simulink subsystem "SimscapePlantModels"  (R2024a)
settings: Solver=VariableStepAuto  StartTime=0.0  StopTime=10.0  RelTol=1e-3
undefined symbols (not defined in the file or in its folder): PlntTrnsfrCaseAxlSpdLock, PlntTrnsfrCaseTrqSplitRatio
libraries: simulink x2, nesl_utility x2

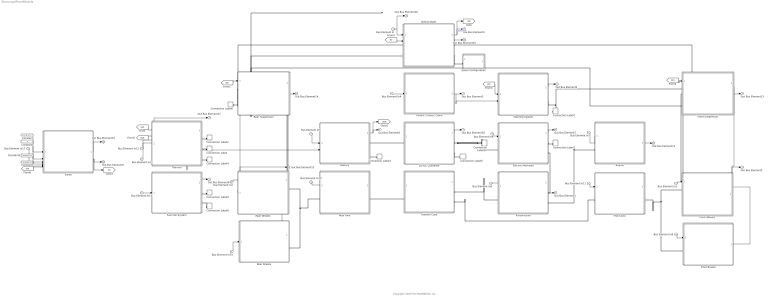
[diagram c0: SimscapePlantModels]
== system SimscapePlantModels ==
  note: Copyright 2023 The MathWorks, Inc.
  Bus Element In{,1..3} (4 alike) : Inport
  Bus Element In4 : Inport  Port=2
  Bus Element In{5..14,17} (11 alike) : Inport  Port=3
  Battery : Subsystem  Variant=on  VariantChoicesSpecifier={'BatteryMappedSSC', 'DetailedBatteryModel', 'NoBattery'}  VariantControlMode=label  VariantControl=Battery  LabelModeActiveChoice=NoBattery
  Connection Label : ConnectionLabel  Label=ThrmEM
  Connection Label1 : ConnectionLabel  Label=ThrmEM
  Connection Label10 : ConnectionLabel  Label=HVDC
  Connection Label2 : ConnectionLabel  Label=ThrmBatt
  Connection Label3 : ConnectionLabel  Label=ThrmBatt
  Connection Label4 : ConnectionLabel  Label=ThrmPwrE
  Connection Label5 : ConnectionLabel  Label=ThrmPwrE
  Connection Label6 : ConnectionLabel  Label=Steer
  Connection Label7 : ConnectionLabel  Label=Steer
  Connection Label8 : ConnectionLabel  Label=ThrmPwrE
  Connection Label9 : ConnectionLabel  Label=HVDC
  Constant : Constant  Value=[0 0 0 0 0 0]
  Constant1 : Constant  Value=0
  Constant3 : Constant  Value=zeros(2,1)
  Constant4 : Constant  Value=ones(2,1)
  DC-DC Converter : Subsystem  Variant=on  VariantChoicesSpecifier={'DCDCConverterSSC', 'HVDCPassThroughSSC', 'NoDCDCConverter'}  VariantControlMode=label  VariantControl=DC-DC Converter  LabelModeActiveChoice=NoDCDCConverter
  Electric Machines : Subsystem  Variant=on  VariantChoicesSpecifier={'s1EMSSC', 's2EMSSC', 's3EMSSC', 's4EMSSC', 'NoEM'}  VariantControlMode=label  VariantControl=Electric Machines  LabelModeActiveChoice=NoEM
  Engine : Subsystem  Variant=on  VariantChoicesSpecifier={'FMUEngineSSC', 'NoEngine', 'SimpleEngineSSC'}  VariantControlMode=label  VariantControl=Engine  LabelModeActiveChoice=SimpleEngineSSC
  Front Axle : Subsystem  Variant=on  VariantChoicesSpecifier={'DualEMDriveFrontSSC', 'LimitedSlipDifferentialSSC', 'NoDifferentialFrontSSC', 'OpenDifferentialSSC'}  VariantControlMode=label  VariantControl=Front Axle  LabelModeActiveChoice=OpenDifferentialSSC
  Front Brakes : Subsystem  Variant=on  VariantControlMode=label  LabelModeActiveChoice=BrakingHydraulicsDiscBrakesFrontSSC
  Front Suspension : Subsystem  Variant=on  VariantChoicesSpecifier={'NoSuspensionFrontSSC', 'MultibodySuspensionFrontSSC'}  VariantControlMode=label  VariantControl=Front Suspension  LabelModeActiveChoice=NoSuspensionFrontSSC
  Front Wheels : Subsystem  Variant=on  VariantChoicesSpecifier={'MFTiresLongitudinalFrontSSC', 'MFTiresMultibodyFrontSSC'}  VariantControlMode=label  VariantControl=Front Wheels  LabelModeActiveChoice=MFTiresLongitudinalFrontSSC
  Fuel Cell System : Subsystem  Variant=on  VariantControlMode=label  LabelModeActiveChoice=NoFuelCell
  "Pedals, Cluster, Cabin" : Subsystem
  Rear Axle : Subsystem  Variant=on  VariantChoicesSpecifier={'DualEMDriveRear3EMSSC', 'DualEMDriveRear4EMSSC', 'LimitedSlipDifferential2SSC', 'NoDifferentialRearSSC', 'OpenDifferential2SSC'}  VariantControlMode=label  VariantControl=Rear Axle  LabelModeActiveChoice=NoDifferentialRearSSC
  Rear Brakes : Subsystem  Variant=on  VariantControlMode=label  LabelModeActiveChoice=BrakingHydraulicsDiscBrakesRearSSC
  Rear Suspension : Subsystem  Variant=on  VariantChoicesSpecifier={'NoSuspensionRearSSC', 'MultibodySuspensionRearSSC'}  VariantControlMode=label  VariantControl=Rear Suspension  LabelModeActiveChoice=NoSuspensionRearSSC
  Rear Wheels : Subsystem  Variant=on  VariantChoicesSpecifier={'MFTiresLongitudinalRearSSC', 'MFTiresMultibodyRearSSC'}  VariantControlMode=label  VariantControl=Rear Wheels  LabelModeActiveChoice=MFTiresLongitudinalRearSSC
  Solver Configuration : Subsystem  Variant=on  VariantControlMode=label  VariantControl=Choice  LabelModeActiveChoice=Solver Configuration
  Steering System : Subsystem  Variant=on  VariantChoicesSpecifier={'NoSteering', 'SteeringSystemSSC'}  VariantControlMode=label  VariantControl=Steering System  LabelModeActiveChoice=NoSteering
  Thermal : Subsystem  Variant=on  VariantChoicesSpecifier={'ElectricalCoolingSystemSSC', 'ElectricalThermalSystemSSC', 'NoThermalEffectSSC'}  VariantControlMode=label  VariantControl=Thermal  LabelModeActiveChoice=NoThermalEffectSSC
  Trailer : Subsystem  Variant=on  VariantChoicesSpecifier={'NoTrailer'}  VariantControlMode=label  VariantControl=No Trailer  LabelModeActiveChoice=NoTrailer
  Transfer Case : Subsystem
  Transmission : Subsystem  Variant=on  VariantChoicesSpecifier={'BEV1EMSSC', 'BEV2EMSSC', 'BEV3EMSSC', 'BEV4EMSSC', 'ConventionalVehicleSSC', 'HEVIPSSSC', 'HEVMMSSC', 'HEVP0SSC', 'HEVP1SSC', 'HEVP2SSC', 'HEVP3SSC', 'HEVP4SSC'}  VariantControlMode=label  VariantControl=Transmission  LabelModeActiveChoice=ConventionalVehicleSSC
  Vehicle Body : Subsystem
  Out Bus Element{1..18} (18 alike) : Outport
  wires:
  "Pedals, Cluster, Cabin"/1(VehFdbk) -> Steering System/2(Driver), Out Bus Element3/1
  Front Wheels/1(FrntWheels) -> Front Suspension/2(FrntWheels), Out Bus Element5/1
  Front Suspension/1(FrntSusp) -> Out Bus Element13/1
  Rear Wheels/1(RearWheels) -> Out Bus Element12/1, Rear Suspension/2(RearWheels)
  Transmission/1(TransInfo) -> Out Bus Element1/1
  Thermal/1(Thermal) -> Out Bus Element17/1, Battery/2(Thermal)
  Bus Element In7/1 -> Engine/1(Cntrl)
  Bus Element In13/1 -> Fuel Cell System/1(Cntrl)
  Engine/1(EngFdbk) -> Out Bus Element11/1
  Vehicle Body/1(Bus Element Out) -> Out Bus Element4/1, [Veh]  "VehFdbk"
  Rear Brakes/1(BrkPrs) -> Rear Wheels/2(BrkPrs)
  Electric Machines/1(EMInfo) -> Out Bus Element7/1
  Steering System/1(Steering) -> Out Bus Element2/1
  Bus Element In2/1 -> Rear Wheels/1(Env)
  Bus Element In/1 -> Vehicle Body/1(Bus Element In), Out Bus Element16/1
  Bus Element In4/1 -> "Pedals, Cluster, Cabin"/1(Driver)
  Bus Element In3/1 -> Thermal/4(Env)
  Bus Element In14/1 -> Rear Brakes/1(Cntrl)
  Front Brakes/1(BrkPrs) -> Front Wheels/2(BrkPrs)
  Bus Element In9/1 -> Transmission/1(Cntrl)
  Bus Element In12/1 -> Thermal/3(Cntrl)
  Bus Element In8/1 -> Front Brakes/1(Cntrl)
  Bus Element In5/1 -> Battery/1(Cntrl)
  Rear Suspension/1(RearSusp) -> Out Bus Element14/1
  Fuel Cell System/1(FuelCell) -> Out Bus Element8/1
  Bus Element In6/1 -> Electric Machines/1(Cntrl)
  Bus Element In1/1 -> Front Wheels/1(Env)
  Battery/1(Battery) -> Out Bus Element6/1, [Batt]
  Bus Element In10/1 -> Rear Axle/1(Cntrl)
  Bus Element In11/1 -> Front Axle/1(Cntrl)
  Vehicle Body/2(Bus Element Out8) -> Out Bus Element15/1
  [Veh] -> Thermal/1(VehBody)
  [Veh] -> Rear Suspension/1(Veh)
  [Veh] -> Front Suspension/1(Veh)
  [Veh] -> Steering System/1(VehSpd)
  [Trlr] -> Vehicle Body/2(Hitch)
  DC-DC Converter/1(DCDC) -> Out Bus Element18/1
  [Batt] -> Thermal/2(Batt)
  Trailer/2(TrlrBody) -> [Trlr], Out Bus Element9/1
  [Veh] -> Trailer/6(Vehicle Hitch)
  Bus Element In17/1 -> Trailer/3(BrkPrs)
  Constant/1 -> Trailer/1(WhlAng)
  Constant3/1 -> Trailer/4(Ground)
  Constant4/1 -> Trailer/5(Friction)
  Constant1/1 -> Trailer/2(AxlTrq)
  Trailer/1(Wheels) -> Out Bus Element10/1
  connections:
  Rear Suspension/LConn2 -- Front Suspension/LConn3 -- Vehicle Body/LConn2
  Rear Brakes/RConn1 -- Rear Wheels/LConn1 -- Rear Axle/RConn1
  Front Brakes/LConn1 -- Front Wheels/LConn1 -- Front Axle/RConn1
  DC-DC Converter/RConn1 -- Electric Machines/LConn1 -- Connection Label10/LConn1
  Connection Label7/LConn1 -- Steering System/RConn1 -- Front Suspension/LConn1
  Fuel Cell System/RConn1 -- Connection Label9/LConn1
  Connection Label8/LConn1 -- Fuel Cell System/RConn2
  Thermal/LConn1 -- Connection Label2/LConn1
  Transmission/LConn1 -- Electric Machines/RConn2
  Front Axle/LConn1 -- Transfer Case/RConn2
  Rear Suspension/LConn3 -- Vehicle Body/LConn1
  Thermal/LConn2 -- Connection Label/LConn1
  Thermal/LConn3 -- Connection Label4/LConn1
  Electric Machines/RConn1 -- Connection Label1/LConn1
  Rear Wheels/LConn3 -- Rear Suspension/RConn1
  Rear Suspension/LConn1 -- Connection Label6/LConn1
  DC-DC Converter/LConn1 -- Battery/RConn1
  Transmission/LConn2 -- Engine/RConn1
  DC-DC Converter/RConn2 -- Connection Label5/LConn1
  Battery/RConn2 -- Connection Label3/LConn1
  Front Wheels/LConn2 -- Front Suspension/RConn1
  Rear Axle/LConn1 -- Transfer Case/LConn1
  Vehicle Body/RConn2 -- Solver Configuration/RConn1
  Vehicle Body/RConn1 -- Front Suspension/LConn2
  Transmission/RConn1 -- Transfer Case/RConn1
  Front Wheels/LConn3 -- Front Suspension/RConn2
  Rear Wheels/LConn2 -- Rear Suspension/RConn2

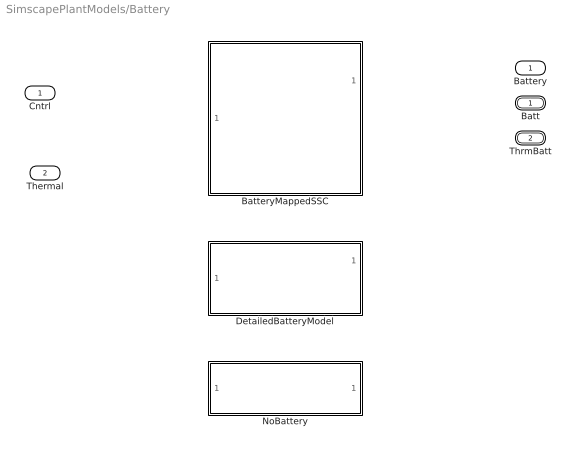
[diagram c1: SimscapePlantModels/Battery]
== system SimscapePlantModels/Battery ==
  Cntrl : Inport
  Thermal : Inport  Port=2
  BatteryMappedSSC : Subsystem  VariantControl=BatteryMappedSSC  ReferencedSubsystem=BatteryMappedSSC
  DetailedBatteryModel : Subsystem  VariantControl=DetailedBatteryModel  ReferencedSubsystem=DetailedBatteryModel
  NoBattery : Subsystem  VariantControl=NoBattery  ReferencedSubsystem=NoBattery
  Batt : PMIOPort  Side=Right
  ThrmBatt : PMIOPort  Port=2  Side=Right
  Battery : Outport

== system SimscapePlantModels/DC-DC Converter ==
  DCDCConverterSSC : Subsystem  VariantControl=DCDCConverterSSC  ReferencedSubsystem=DCDCConverterSSC
  HVDCPassThroughSSC : Subsystem  VariantControl=HVDCPassThroughSSC  ReferencedSubsystem=HVDCPassThroughSSC
  NoDCDCConverter : Subsystem  VariantControl=NoDCDCConverter  ReferencedSubsystem=NoDCDCConverter
  Batt : PMIOPort  Side=Left
  HVDC : PMIOPort  Port=2  Side=Right
  ThrmPwrE : PMIOPort  Port=3  Side=Right
  DCDC : Outport

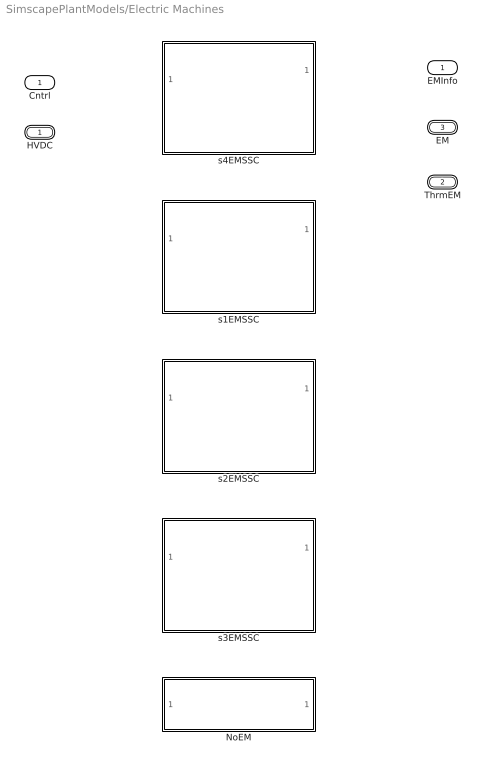
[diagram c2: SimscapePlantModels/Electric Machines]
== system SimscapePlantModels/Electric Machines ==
  Cntrl : Inport
  NoEM : Subsystem  VariantControl=NoEM  ReferencedSubsystem=NoEM
  s1EMSSC : Subsystem  VariantControl=s1EMSSC  ReferencedSubsystem=s1EMSSC
  s2EMSSC : Subsystem  VariantControl=s2EMSSC  ReferencedSubsystem=s2EMSSC
  s3EMSSC : Subsystem  VariantControl=s3EMSSC  ReferencedSubsystem=s3EMSSC
  s4EMSSC : Subsystem  VariantControl=s4EMSSC  ReferencedSubsystem=s4EMSSC
  HVDC : PMIOPort  Side=Left
  ThrmEM : PMIOPort  Port=2  Side=Right
  EM : PMIOPort  Port=3  Side=Right
  EMInfo : Outport

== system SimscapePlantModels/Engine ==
  Cntrl : Inport
  FMUEngineSSC : Subsystem  VariantControl=FMUEngineSSC  ReferencedSubsystem=FMUEngineSSC
  NoEngine : Subsystem  VariantControl=NoEngine  ReferencedSubsystem=NoEngine
  SimpleEngineSSC : Subsystem  VariantControl=SimpleEngineSSC  ReferencedSubsystem=SimpleEngineSSC
  EngTrq : PMIOPort  Side=Right
  EngFdbk : Outport

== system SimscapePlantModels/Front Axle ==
  Cntrl : Inport
  DualEMDriveFrontSSC : Subsystem  VariantControl=DualEMDriveFrontSSC  ReferencedSubsystem=DualEMDriveFrontSSC
  LimitedSlipDifferentialSSC : Subsystem  VariantControl=LimitedSlipDifferentialSSC  ReferencedSubsystem=LimitedSlipDifferentialSSC
  NoDifferentialFrontSSC : Subsystem  VariantControl=NoDifferentialFrontSSC  ReferencedSubsystem=NoDifferentialFrontSSC
  OpenDifferentialSSC : Subsystem  VariantControl=OpenDifferentialSSC  ReferencedSubsystem=OpenDifferentialSSC
  DriveshftTrq : PMIOPort  Side=Left
  AxlTrq : PMIOPort  Port=2  Side=Right

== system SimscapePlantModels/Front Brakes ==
  Cntrl : Inport
  BrakingHydraulicsDiscBrakesFrontSSC : Subsystem  VariantControl=BrakingHydraulicsDiscBrakesFrontSSC  ReferencedSubsystem=BrakingHydraulicsDiscBrakesFrontSSC
  Axl : PMIOPort  Side=Left
  BrkPrs : Outport

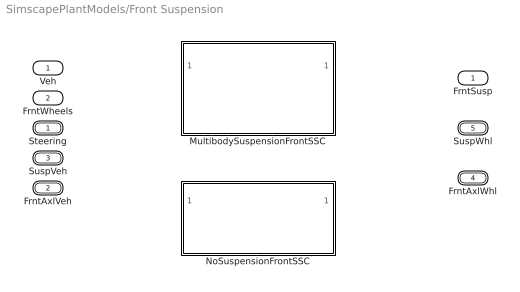
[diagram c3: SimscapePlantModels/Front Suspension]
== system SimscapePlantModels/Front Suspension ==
  Veh : Inport
  FrntWheels : Inport  Port=2
  MultibodySuspensionFrontSSC : Subsystem  VariantControl=MultibodySuspensionFrontSSC  ReferencedSubsystem=MultibodySuspensionFrontSSC
  NoSuspensionFrontSSC : Subsystem  VariantControl=NoSuspensionFrontSSC  ReferencedSubsystem=NoSuspensionFrontSSC
  Steering : PMIOPort  Side=Left
  FrntAxlVeh : PMIOPort  Port=2  Side=Left
  SuspVeh : PMIOPort  Port=3  Side=Left
  FrntAxlWhl : PMIOPort  Port=4  Side=Right
  SuspWhl : PMIOPort  Port=5  Side=Right
  FrntSusp : Outport

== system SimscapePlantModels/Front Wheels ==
  Env : Inport
  BrkPrs : Inport  Port=2
  MFTiresLongitudinalFrontSSC : Subsystem  VariantControl=MFTiresLongitudinalFrontSSC  ReferencedSubsystem=MFTiresLongitudinalFrontSSC
  MFTiresMultibodyFrontSSC : Subsystem  VariantControl=MFTiresMultibodyFrontSSC  ReferencedSubsystem=MFTiresMultibodyFrontSSC
  Axl : PMIOPort  Side=Left
  FrntAxlWhl : PMIOPort  Port=2  Side=Left
  SuspWhl : PMIOPort  Port=3  Side=Left
  FrntWheels : Outport

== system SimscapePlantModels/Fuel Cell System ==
  Cntrl : Inport
  FuelCellSSC : Subsystem  VariantControl=FuelCellSSC  ReferencedSubsystem=FuelCellSSC
  NoFuelCell : Subsystem  VariantControl=NoFuelCell  ReferencedSubsystem=NoFuelCell
  HVDC : PMIOPort  Side=Right
  H : PMIOPort  Port=2  Side=Right
  FuelCell : Outport

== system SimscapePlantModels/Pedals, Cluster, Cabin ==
  Driver : Inport
  Pedal Cluster Input : Subsystem
  "Pedal, Cluster, Cabin" : Subsystem
  VehFdbk : Outport
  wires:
  Pedal Cluster Input/1(SteerCmd) -> "Pedal, Cluster, Cabin"/1(SteerCmd)
  Pedal Cluster Input/2(AccelCmd) -> "Pedal, Cluster, Cabin"/2(AccCmd)
  Pedal Cluster Input/3(DecelCmd) -> "Pedal, Cluster, Cabin"/3(DecelCmd)
  Pedal Cluster Input/4(DrvrGearCmd) -> "Pedal, Cluster, Cabin"/4(GearCmd)
  Pedal Cluster Input/5(IgnCmd) -> "Pedal, Cluster, Cabin"/5(IgCmd)
  Pedal Cluster Input/6(HighBeamCmd) -> "Pedal, Cluster, Cabin"/6(HighBeamCmd)
  Pedal Cluster Input/7(LowBeamCmd) -> "Pedal, Cluster, Cabin"/7(LowBeamCmd)
  Pedal Cluster Input/8(LeftSignalCmd) -> "Pedal, Cluster, Cabin"/8(LeftSignalCmd)
  Pedal Cluster Input/9(RightSignalCmd) -> "Pedal, Cluster, Cabin"/9(RightSignalCmd)
  Pedal Cluster Input/10(HazzardCmd) -> "Pedal, Cluster, Cabin"/10(HazzardCmd)
  Driver/1 -> Pedal Cluster Input/1(Driver)
  "Pedal, Cluster, Cabin"/1(Driver) -> VehFdbk/1

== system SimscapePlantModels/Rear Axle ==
  Cntrl : Inport
  DualEMDriveRear3EMSSC : Subsystem  VariantControl=DualEMDriveRear3EMSSC  ReferencedSubsystem=DualEMDriveRear3EMSSC
  DualEMDriveRear4EMSSC : Subsystem  VariantControl=DualEMDriveRear4EMSSC  ReferencedSubsystem=DualEMDriveRear4EMSSC
  LimitedSlipDifferential2SSC : Subsystem  VariantControl=LimitedSlipDifferential2SSC  ReferencedSubsystem=LimitedSlipDifferential2SSC
  NoDifferentialRearSSC : Subsystem  VariantControl=NoDifferentialRearSSC  ReferencedSubsystem=NoDifferentialRearSSC
  OpenDifferential2SSC : Subsystem  VariantControl=OpenDifferential2SSC  ReferencedSubsystem=OpenDifferential2SSC
  DriveshftTrq : PMIOPort  Side=Left
  AxlTrq : PMIOPort  Port=2  Side=Right

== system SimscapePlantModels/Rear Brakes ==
  Cntrl : Inport
  BrakingHydraulicsDiscBrakesRearSSC : Subsystem  VariantControl=BrakingHydraulicsDiscBrakesRearSSC  ReferencedSubsystem=BrakingHydraulicsDiscBrakesRearSSC
  Axl : PMIOPort  Side=Right
  BrkPrs : Outport

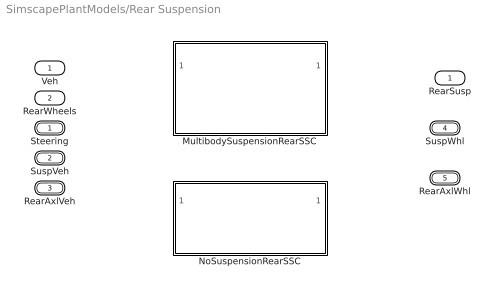
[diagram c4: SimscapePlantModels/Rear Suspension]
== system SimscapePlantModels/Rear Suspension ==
  Veh : Inport
  RearWheels : Inport  Port=2
  MultibodySuspensionRearSSC : Subsystem  VariantControl=MultibodySuspensionRearSSC  ReferencedSubsystem=MultibodySuspensionRearSSC
  NoSuspensionRearSSC : Subsystem  VariantControl=NoSuspensionRearSSC  ReferencedSubsystem=NoSuspensionRearSSC
  Steering : PMIOPort  Side=Left
  SuspVeh : PMIOPort  Port=2  Side=Left
  RearAxlVeh : PMIOPort  Port=3  Side=Left
  SuspWhl : PMIOPort  Port=4  Side=Right
  RearAxlWhl : PMIOPort  Port=5  Side=Right
  RearSusp : Outport

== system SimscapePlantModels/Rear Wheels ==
  Env : Inport
  BrkPrs : Inport  Port=2
  MFTiresLongitudinalRearSSC : Subsystem  VariantControl=MFTiresLongitudinalRearSSC  ReferencedSubsystem=MFTiresLongitudinalRearSSC
  MFTiresMultibodyRearSSC : Subsystem  VariantControl=MFTiresMultibodyRearSSC  ReferencedSubsystem=MFTiresMultibodyRearSSC
  Axl : PMIOPort  Side=Left
  RearAxlWhl : PMIOPort  Port=2  Side=Left
  SuspWhl : PMIOPort  Port=3  Side=Left
  RearWheels : Outport

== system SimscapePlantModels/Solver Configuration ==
  Local Solver : nesl_utility/Solver Configuration  VariantControl=Local Solver  PhysicalDomain=network_engine_domain  SubClassName=solver  LeftPortType=input  RightPortType=generic  Tones=[]  Harmonics=[]  SimulateNoise=off  Profile=off  UseLocalSampling=off  EnableSwitchedLinearOptims=on  FrequencyDomain=off  UseCCode=off  RelTol=0.001  AbsTol=0.001  MinStep=1e-09  ToWorkspace=off  RevertToSquareIcSolve=off  NumHomotopyIterations=100  PhasorMode=off  PhasorModeNumHarmonics=1  ConsistencySolver=NEWTON_XTOL_AFTER_FTOL  IndexReductionMethod=DerivativeReplacement  DoDC=off  ResidualTolerance=1e-09  ConsistencyTolSource=LOCAL  ConsistencyAbsTol=0.001  ConsistencyRelTol=0.001  ConsistencyTolFactor=0.001  UseLocalSolver=on  LocalSolverChoice=NE_BACKWARD_EULER_ADVANCER  ResolveIndetEquations=on  FunctionEvalNumThread=1  LocalSolverSampleTime=0.1  DoFixedCost=off  MaxNonlinIter=3  MaxModeIter=2  ComputeImpulses=off  ImpulseIterations=2  LinearAlgebra=auto  LinearAlgebraNumThread=0  EquationFormulation=NE_TIME_EF  DelaysMemoryBudget=1024  AutomaticFiltering=on  FilteringTimeConstant=0.001  PartitionStorageMethod=AS_NEEDED  PartitionMemoryBudget=1024  PartitionMethod=ROBUST  MultibodyUseLocalSolver=off  MultibodyLocalSolverChoice=ODE1  MultibodyLocalSolverSampleTime=0.001
  Solver Configuration : nesl_utility/Solver Configuration  VariantControl=Solver Configuration  PhysicalDomain=network_engine_domain  SubClassName=solver  LeftPortType=input  RightPortType=generic  Tones=[]  Harmonics=[]  SimulateNoise=off  Profile=off  UseLocalSampling=off  EnableSwitchedLinearOptims=on  FrequencyDomain=off  UseCCode=off  RelTol=0.001  AbsTol=0.001  MinStep=1e-09  ToWorkspace=off  RevertToSquareIcSolve=off  NumHomotopyIterations=100  PhasorMode=off  PhasorModeNumHarmonics=1  ConsistencySolver=NEWTON_XTOL_AFTER_FTOL  IndexReductionMethod=DerivativeReplacement  DoDC=off  ResidualTolerance=1e-09  ConsistencyTolSource=LOCAL  ConsistencyAbsTol=0.001  ConsistencyRelTol=0.001  ConsistencyTolFactor=0.001  UseLocalSolver=off  LocalSolverChoice=NE_BACKWARD_EULER_ADVANCER  ResolveIndetEquations=on  FunctionEvalNumThread=1  LocalSolverSampleTime=0.001  DoFixedCost=off  MaxNonlinIter=3  MaxModeIter=2  ComputeImpulses=off  ImpulseIterations=2  LinearAlgebra=auto  LinearAlgebraNumThread=0  EquationFormulation=NE_TIME_EF  DelaysMemoryBudget=1024  AutomaticFiltering=on  FilteringTimeConstant=0.001  PartitionStorageMethod=AS_NEEDED  PartitionMemoryBudget=1024  PartitionMethod=ROBUST  MultibodyUseLocalSolver=off  MultibodyLocalSolverChoice=ODE1  MultibodyLocalSolverSampleTime=0.001
  a : PMIOPort  Side=Right

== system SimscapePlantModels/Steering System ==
  VehSpd : Inport
  Driver : Inport  Port=2
  NoSteering : Subsystem  VariantControl=NoSteering  ReferencedSubsystem=NoSteering
  SteeringSystemSSC : Subsystem  VariantControl=SteeringSystemSSC  ReferencedSubsystem=SteeringSystemSSC
  SteerSusp : PMIOPort  Side=Right
  Steering : Outport

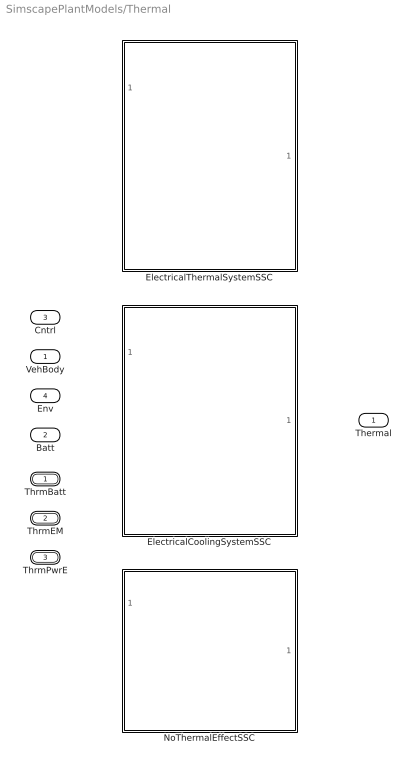
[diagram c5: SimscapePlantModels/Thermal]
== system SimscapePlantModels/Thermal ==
  VehBody : Inport
  Batt : Inport  Port=2
  Cntrl : Inport  Port=3
  Env : Inport  Port=4
  ElectricalCoolingSystemSSC : Subsystem  VariantControl=ElectricalCoolingSystemSSC  ReferencedSubsystem=ElectricalCoolingSystemSSC
  ElectricalThermalSystemSSC : Subsystem  VariantControl=ElectricalThermalSystemSSC  ReferencedSubsystem=ElectricalThermalSystemSSC
  NoThermalEffectSSC : Subsystem  VariantControl=NoThermalEffectSSC  ReferencedSubsystem=NoThermalEffectSSC
  ThrmBatt : PMIOPort  Side=Left
  ThrmEM : PMIOPort  Port=2  Side=Left
  ThrmPwrE : PMIOPort  Port=3  Side=Left
  Thermal : Outport

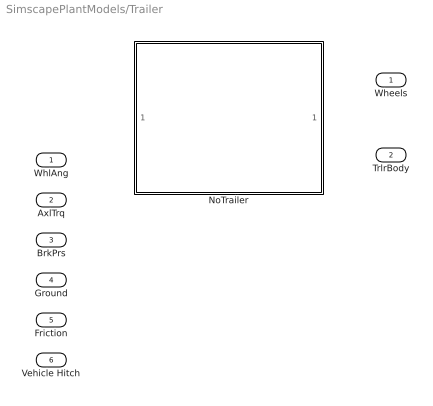
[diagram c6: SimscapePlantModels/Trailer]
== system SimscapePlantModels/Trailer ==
  WhlAng : Inport
  AxlTrq : Inport  Port=2
  BrkPrs : Inport  Port=3
  Ground : Inport  Port=4
  Friction : Inport  Port=5
  Vehicle Hitch : Inport  Port=6
  NoTrailer : Subsystem  VariantControl=NoTrailer  ReferencedSubsystem=NoTrailer
  Wheels : Outport
  TrlrBody : Outport  Port=2

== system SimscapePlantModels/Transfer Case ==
  Axle Interconnect : Subsystem  Variant=on  VariantChoicesSpecifier={'NoInterconnectSSC', 'TransferCaseSSC'}  VariantControlMode=label  VariantControl=Choice  LabelModeActiveChoice=NoInterconnectSSC
  Constant : Constant  Value=PlntTrnsfrCaseTrqSplitRatio  SampleTime=-1
  Constant1 : Constant  Value=PlntTrnsfrCaseAxlSpdLock  SampleTime=-1
  DriveshftTrq Routing : Subsystem  Variant=on  VariantChoicesSpecifier={'FourActuatorAWDSSC', 'OneActuatorAWDSSC', 'OneActuatorFWDSSC', 'OneActuatorRWDSSC', 'ThreeActuatorAWD2EMFrontSSC', 'ThreeActuatorAWD2EMRearSSC', 'TwoActuatorAWDSSC'}  VariantControlMode=label  VariantControl=Choice  LabelModeActiveChoice=OneActuatorFWDSSC
  Terminator : Terminator
  DriveshftTrq : PMIOPort  Side=Right
  FrntDiffrntlTrq : PMIOPort  Port=2  Side=Right
  RearDiffrntlTrq : PMIOPort  Port=3  Side=Left
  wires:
  DriveshftTrq Routing/1(DriveshftSpd) -> Terminator/1
  Constant1/1 -> Axle Interconnect/2(Lockup)
  Constant/1 -> Axle Interconnect/1(SplitRatio)
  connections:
  RearDiffrntlTrq/RConn1 -- DriveshftTrq Routing/RConn5
  Axle Interconnect/LConn2 -- DriveshftTrq Routing/RConn3
  Axle Interconnect/LConn3 -- DriveshftTrq Routing/RConn4
  Axle Interconnect/LConn1 -- DriveshftTrq Routing/RConn2
  DriveshftTrq/RConn1 -- DriveshftTrq Routing/LConn1
  DriveshftTrq Routing/RConn1 -- FrntDiffrntlTrq/RConn1

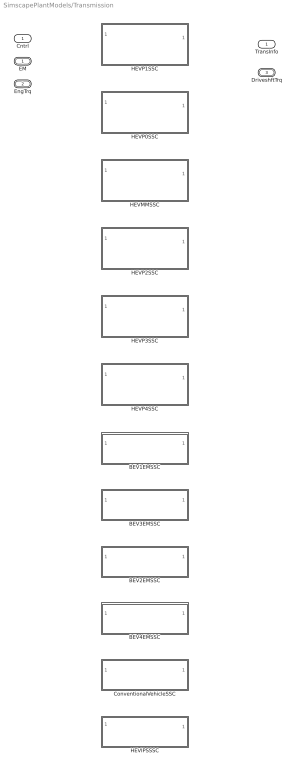
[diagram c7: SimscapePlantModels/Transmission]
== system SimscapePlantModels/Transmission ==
  Cntrl : Inport
  BEV1EMSSC : Subsystem  VariantControl=BEV1EMSSC  ReferencedSubsystem=BEV1EMSSC
  BEV2EMSSC : Subsystem  VariantControl=BEV2EMSSC  ReferencedSubsystem=BEV2EMSSC
  BEV3EMSSC : Subsystem  VariantControl=BEV3EMSSC  ReferencedSubsystem=BEV3EMSSC
  BEV4EMSSC : Subsystem  VariantControl=BEV4EMSSC  ReferencedSubsystem=BEV4EMSSC
  ConventionalVehicleSSC : Subsystem  VariantControl=ConventionalVehicleSSC  ReferencedSubsystem=ConventionalVehicleSSC
  HEVIPSSSC : Subsystem  VariantControl=HEVIPSSSC  ReferencedSubsystem=HEVIPSSSC
  HEVMMSSC : Subsystem  VariantControl=HEVMMSSC  ReferencedSubsystem=HEVMMSSC
  HEVP0SSC : Subsystem  VariantControl=HEVP0SSC  ReferencedSubsystem=HEVP0SSC
  HEVP1SSC : Subsystem  VariantControl=HEVP1SSC  ReferencedSubsystem=HEVP1SSC
  HEVP2SSC : Subsystem  VariantControl=HEVP2SSC  ReferencedSubsystem=HEVP2SSC
  HEVP3SSC : Subsystem  VariantControl=HEVP3SSC  ReferencedSubsystem=HEVP3SSC
  HEVP4SSC : Subsystem  VariantControl=HEVP4SSC  ReferencedSubsystem=HEVP4SSC
  EM : PMIOPort  Side=Left
  EngTrq : PMIOPort  Port=2  Side=Left
  DriveshftTrq : PMIOPort  Port=3  Side=Right
  TransInfo : Outport

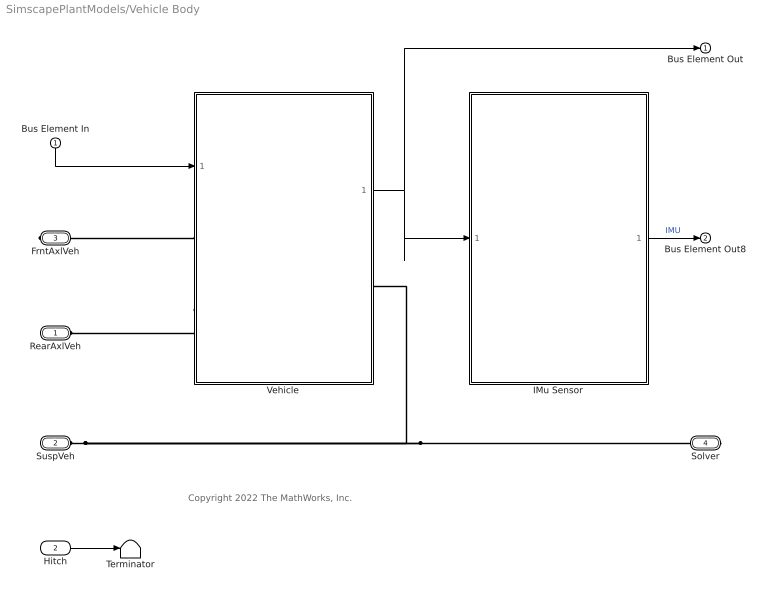
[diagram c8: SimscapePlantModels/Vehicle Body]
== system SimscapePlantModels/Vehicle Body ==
  note: Copyright 2022 The MathWorks, Inc.
  Bus Element In : Inport
  Hitch : Inport  Port=2
  IMu Sensor : Subsystem  Variant=on  VariantChoicesSpecifier={'IMUSensor', 'NoIMUSensor'}  VariantControlMode=label  VariantControl=Choice  LabelModeActiveChoice=NoIMUSensor
  Terminator : Terminator
  Vehicle : Subsystem  Variant=on  VariantChoicesSpecifier={'VehicleBody1DOFLongitudinalSSC', 'VehicleBody3DOFLongitudinalSSC', 'VehicleBody6DOFSSC'}  VariantControlMode=label  VariantControl=Vehicle  LabelModeActiveChoice=VehicleBody3DOFLongitudinalSSC
  RearAxlVeh : PMIOPort  Side=Left
  SuspVeh : PMIOPort  Port=2  Side=Left
  FrntAxlVeh : PMIOPort  Port=3  Side=Right
  Solver : PMIOPort  Port=4  Side=Right
  Bus Element Out : Outport
  Bus Element Out8 : Outport  Port=2
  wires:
  Hitch/1 -> Terminator/1
  Vehicle/1(VehBody) -> IMu Sensor/1(Veh), Bus Element Out/1
  Bus Element In/1 -> Vehicle/1(Env)
  IMu Sensor/1(IMU) -> Bus Element Out8/1  "IMU"
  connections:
  SuspVeh/RConn1 -- Solver/RConn1 -- Vehicle/RConn1
  Vehicle/LConn2 -- RearAxlVeh/RConn1
  Vehicle/LConn1 -- FrntAxlVeh/RConn1

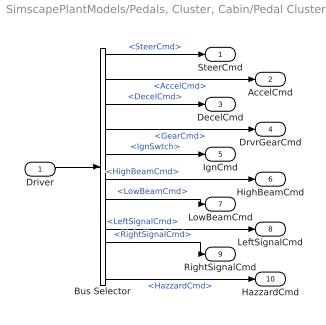
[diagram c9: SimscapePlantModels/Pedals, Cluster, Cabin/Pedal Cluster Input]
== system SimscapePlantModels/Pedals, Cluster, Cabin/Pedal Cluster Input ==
  Driver : Inport
  Bus Selector : BusSelector  OutputSignals=SteerCmd,AccelCmd,DecelCmd,GearCmd,IgnSwtch,LightsCmd.HighBeamCmd,LightsCmd.LowBeamCmd,LightsCmd.LeftSignalCmd,LightsCmd.RightSignalCmd,LightsCmd.HazzardCmd
  SteerCmd : Outport  VectorParamsAs1DForOutWhenUnconnected=off
  AccelCmd : Outport  Port=2  VectorParamsAs1DForOutWhenUnconnected=off
  DecelCmd : Outport  Port=3  VectorParamsAs1DForOutWhenUnconnected=off
  DrvrGearCmd : Outport  Port=4  VectorParamsAs1DForOutWhenUnconnected=off
  IgnCmd : Outport  Port=5  VectorParamsAs1DForOutWhenUnconnected=off
  HighBeamCmd : Outport  Port=6  VectorParamsAs1DForOutWhenUnconnected=off
  LowBeamCmd : Outport  Port=7  VectorParamsAs1DForOutWhenUnconnected=off
  LeftSignalCmd : Outport  Port=8  VectorParamsAs1DForOutWhenUnconnected=off
  RightSignalCmd : Outport  Port=9  VectorParamsAs1DForOutWhenUnconnected=off
  HazzardCmd : Outport  Port=10  VectorParamsAs1DForOutWhenUnconnected=off
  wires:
  Bus Selector/10 -> HazzardCmd/1  "<HazzardCmd>"
  Bus Selector/9 -> RightSignalCmd/1  "<RightSignalCmd>"
  Bus Selector/8 -> LeftSignalCmd/1  "<LeftSignalCmd>"
  Bus Selector/7 -> LowBeamCmd/1  "<LowBeamCmd>"
  Bus Selector/6 -> HighBeamCmd/1  "<HighBeamCmd>"
  Bus Selector/5 -> IgnCmd/1  "<IgnSwtch>"
  Bus Selector/1 -> SteerCmd/1  "<SteerCmd>"
  Bus Selector/4 -> DrvrGearCmd/1  "<GearCmd>"
  Bus Selector/3 -> DecelCmd/1  "<DecelCmd>"
  Driver/1 -> Bus Selector/1
  Bus Selector/2 -> AccelCmd/1  "<AccelCmd>"

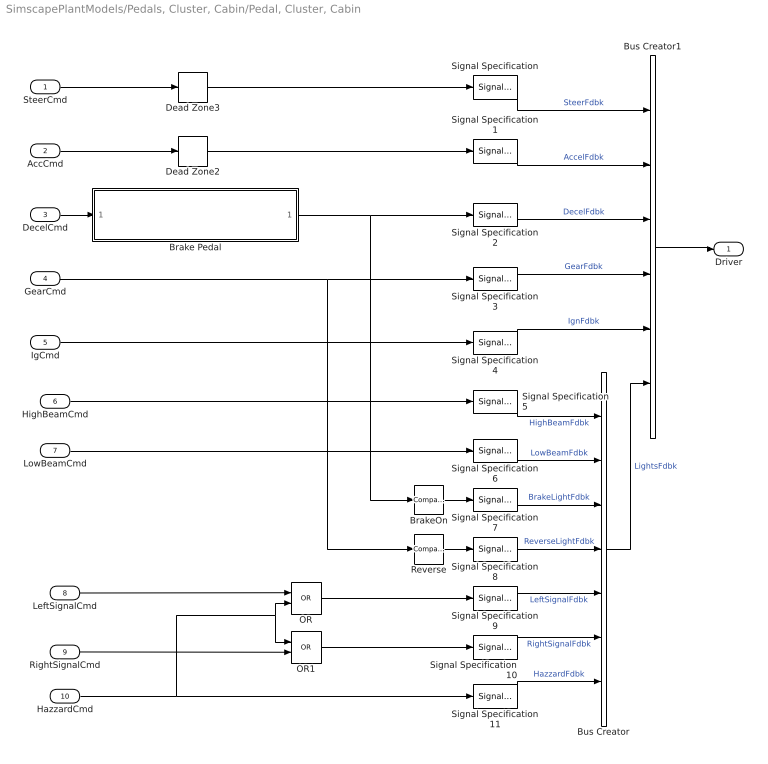
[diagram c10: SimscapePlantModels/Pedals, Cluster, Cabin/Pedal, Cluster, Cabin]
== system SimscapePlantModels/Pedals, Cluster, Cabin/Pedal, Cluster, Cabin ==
  SteerCmd : Inport
  AccCmd : Inport  Port=2
  DecelCmd : Inport  Port=3
  GearCmd : Inport  Port=4
  IgCmd : Inport  Port=5
  HighBeamCmd : Inport  Port=6
  LowBeamCmd : Inport  Port=7
  LeftSignalCmd : Inport  Port=8
  RightSignalCmd : Inport  Port=9
  HazzardCmd : Inport  Port=10
  Brake Pedal : Subsystem
  BrakeOn : simulink/Logic and Bit Operations/Compare To Constant  relop=>  const=0  OutDataTypeStr=boolean  ZeroCross=off
  Bus Creator : BusCreator  Inputs=7
  Bus Creator1 : BusCreator  Inputs=6
  Dead Zone2 : DeadZone  LowerValue=0  UpperValue=.01  ZeroCross=off
  Dead Zone3 : DeadZone  LowerValue=-.01  UpperValue=.01  ZeroCross=off
  OR : Logic  Operator=OR  IconShape=distinctive  AllPortsSameDT=off  OutDataTypeStr=boolean
  OR1 : Logic  Operator=OR  IconShape=distinctive  AllPortsSameDT=off  OutDataTypeStr=boolean
  Reverse : simulink/Logic and Bit Operations/Compare To Constant  relop=<  const=0  OutDataTypeStr=boolean  ZeroCross=off
  Signal Specification : SignalSpecification  Unit=rad
  Signal Specification{1..11} (11 alike) : SignalSpecification  Unit=1
  Driver : Outport
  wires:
  Signal Specification9/1 -> Bus Creator/5  "LeftSignalFdbk"
  Signal Specification11/1 -> Bus Creator/7  "HazzardFdbk"
  Signal Specification10/1 -> Bus Creator/6  "RightSignalFdbk"
  Signal Specification8/1 -> Bus Creator/4  "ReverseLightFdbk"
  Signal Specification7/1 -> Bus Creator/3  "BrakeLightFdbk"
  Signal Specification6/1 -> Bus Creator/2  "LowBeamFdbk"
  Signal Specification5/1 -> Bus Creator/1  "HighBeamFdbk"
  Bus Creator/1 -> Bus Creator1/6  "LightsFdbk"
  RightSignalCmd/1 -> OR1/2
  LowBeamCmd/1 -> Signal Specification6/1
  HazzardCmd/1 -> OR1/1, OR/2, Signal Specification11/1
  LeftSignalCmd/1 -> OR/1
  Reverse/1 -> Signal Specification8/1
  OR/1 -> Signal Specification9/1
  OR1/1 -> Signal Specification10/1
  BrakeOn/1 -> Signal Specification7/1
  HighBeamCmd/1 -> Signal Specification5/1
  Dead Zone3/1 -> Signal Specification/1
  Signal Specification1/1 -> Bus Creator1/2  "AccelFdbk"
  Signal Specification4/1 -> Bus Creator1/5  "IgnFdbk"
  Brake Pedal/1(DecelFdbk) -> Signal Specification2/1, BrakeOn/1
  Signal Specification/1 -> Bus Creator1/1  "SteerFdbk"
  Signal Specification2/1 -> Bus Creator1/3  "DecelFdbk"
  GearCmd/1 -> Signal Specification3/1, Reverse/1
  Bus Creator1/1 -> Driver/1
  IgCmd/1 -> Signal Specification4/1
  Signal Specification3/1 -> Bus Creator1/4  "GearFdbk"
  Dead Zone2/1 -> Signal Specification1/1
  SteerCmd/1 -> Dead Zone3/1
  AccCmd/1 -> Dead Zone2/1
  DecelCmd/1 -> Brake Pedal/1(DecelCmd)

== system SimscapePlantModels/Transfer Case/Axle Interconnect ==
  SplitRatio : Inport
  Lockup : Inport  Port=2
  NoInterconnectSSC : Subsystem  VariantControl=NoInterconnectSSC  ReferencedSubsystem=NoInterconnectSSC
  TransferCaseSSC : Subsystem  VariantControl=TransferCaseSSC  ReferencedSubsystem=TransferCaseSSC
  FrntDiffrntlTrq : PMIOPort  Side=Left
  DriveshftTrq : PMIOPort  Port=2  Side=Left
  RearDiffrntlTrq : PMIOPort  Port=3  Side=Left

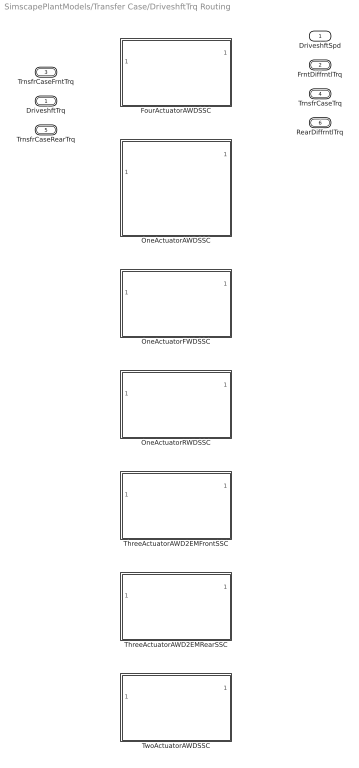
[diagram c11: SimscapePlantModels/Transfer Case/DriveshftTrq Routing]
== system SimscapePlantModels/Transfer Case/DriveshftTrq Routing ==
  FourActuatorAWDSSC : Subsystem  VariantControl=FourActuatorAWDSSC  ReferencedSubsystem=FourActuatorAWDSSC
  OneActuatorAWDSSC : Subsystem  VariantControl=OneActuatorAWDSSC  ReferencedSubsystem=OneActuatorAWDSSC
  OneActuatorFWDSSC : Subsystem  VariantControl=OneActuatorFWDSSC  ReferencedSubsystem=OneActuatorFWDSSC
  OneActuatorRWDSSC : Subsystem  VariantControl=OneActuatorRWDSSC  ReferencedSubsystem=OneActuatorRWDSSC
  ThreeActuatorAWD2EMFrontSSC : Subsystem  VariantControl=ThreeActuatorAWD2EMFrontSSC  ReferencedSubsystem=ThreeActuatorAWD2EMFrontSSC
  ThreeActuatorAWD2EMRearSSC : Subsystem  VariantControl=ThreeActuatorAWD2EMRearSSC  ReferencedSubsystem=ThreeActuatorAWD2EMRearSSC
  TwoActuatorAWDSSC : Subsystem  VariantControl=TwoActuatorAWDSSC  ReferencedSubsystem=TwoActuatorAWDSSC
  DriveshftTrq : PMIOPort  Side=Left
  FrntDiffrntlTrq : PMIOPort  Port=2  Side=Right
  TrnsfrCaseFrntTrq : PMIOPort  Port=3  Side=Right
  TrnsfrCaseTrq : PMIOPort  Port=4  Side=Right
  TrnsfrCaseRearTrq : PMIOPort  Port=5  Side=Right
  RearDiffrntlTrq : PMIOPort  Port=6  Side=Right
  DriveshftSpd : Outport  VectorParamsAs1DForOutWhenUnconnected=off

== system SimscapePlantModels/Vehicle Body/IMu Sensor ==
  Veh : Inport
  IMUSensor : Subsystem  VariantControl=IMUSensor  ReferencedSubsystem=IMUSensor
  NoIMUSensor : Subsystem  VariantControl=NoIMUSensor  ReferencedSubsystem=NoIMUSensor
  IMU : Outport

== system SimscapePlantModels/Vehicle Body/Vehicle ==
  Env : Inport
  VehicleBody1DOFLongitudinalSSC : Subsystem  VariantControl=VehicleBody1DOFLongitudinalSSC  ReferencedSubsystem=VehicleBody1DOFLongitudinalSSC
  VehicleBody3DOFLongitudinalSSC : Subsystem  VariantControl=VehicleBody3DOFLongitudinalSSC  ReferencedSubsystem=VehicleBody3DOFLongitudinalSSC
  VehicleBody6DOFSSC : Subsystem  VariantControl=VehicleBody6DOFSSC  ReferencedSubsystem=VehicleBody6DOFSSC
  FrntAxlVeh : PMIOPort  Side=Left
  RearAxlVeh : PMIOPort  Port=2  Side=Left
  Solver : PMIOPort  Port=3  Side=Right
  VehBody : Outport

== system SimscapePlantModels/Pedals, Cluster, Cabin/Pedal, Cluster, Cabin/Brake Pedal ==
  DecelCmd : Inport
  Dead Zone1 : DeadZone  LowerValue=0  UpperValue=.01  ZeroCross=off
  DecelFdbk : Outport
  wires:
  Dead Zone1/1 -> DecelFdbk/1
  DecelCmd/1 -> Dead Zone1/1
